(* =======================================================================================================================================
   OOP: Extended sample
   =======================================================================================================================================
   Description: 
   This PLC sample contains an object-oriented program to control a sorting system.
   The application can be controlled via an integrated visualization.
   
   PLC_SortingSystem_PLC:
   The functionality of the sorting system is implemented within this PLC project (PLC_SortingSystem_PLC).
   It also contains the visualization to control the application.
   
   PLC_SortingSystem_Simu:
   To run the project without hardware, the simulation PLC can be used.
   For example, It simulates the cylinder positions and temperatures, as well as the sensor signals (correspondent to the box positions). 
   =======================================================================================================================================
   InfoSys:
   https://infosys.beckhoff.de/content/1033/tc3_sampleprogram1/45035996374683915.html?id=6126826020926170206
   https://infosys.beckhoff.de/content/1033/tc3_plc_intro/72057596565231755.html?id=3937754078542861062
   ======================================================================================================================================= *)
PROGRAM MAIN_Simu
VAR

	Simulation	: FB_Simulation;
	
END_VAR

Simulation();

END_PROGRAM
